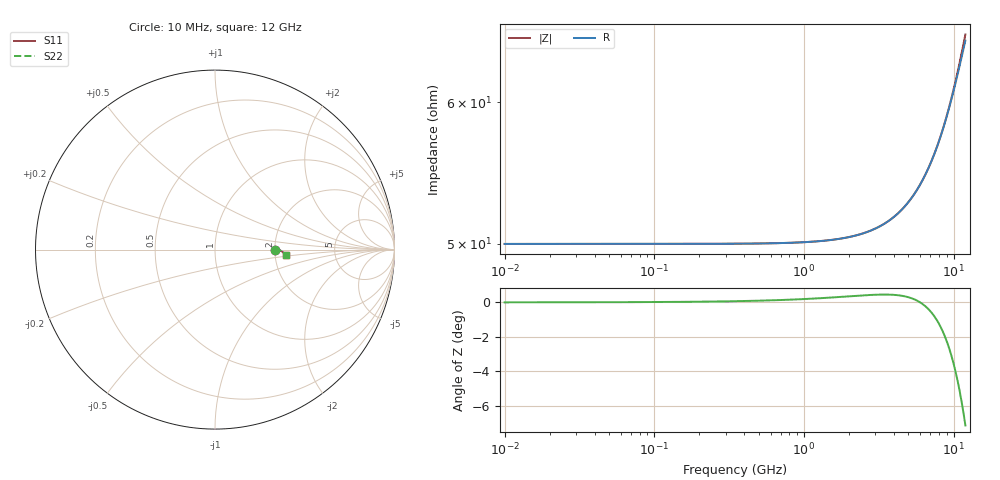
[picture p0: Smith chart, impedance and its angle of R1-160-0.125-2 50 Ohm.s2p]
!version-2
!date-03.2021
# MHz S RI R 50
!Freq ReS11 ImS11 ReS21 ImS21 ReS12 ImS12 ReS22 ImS22
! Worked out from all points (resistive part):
!   601 points, 10 MHz to 12 GHz, reference 50 ohm
!   read as one part in series: R = 50 ohm at 70 MHz
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10  0.3333 7.68e-06  0.6667 -7.7e-06  0.6667 -7.7e-06  0.3333 7.67e-06
510  0.3335 0.000389  0.6665 -0.00039  0.6665 -0.00039  0.3335 0.000388
1010  0.3338 0.000754  0.6662 -0.000755  0.6662 -0.000755  0.3338 0.000753
1510  0.3345 0.00109  0.6655 -0.00109  0.6655 -0.00109  0.3345 0.00109
2010  0.3353 0.00137  0.6647 -0.00138  0.6647 -0.00138  0.3353 0.00137
2510  0.3364 0.00159  0.6636 -0.0016  0.6636 -0.0016  0.3364 0.00159
3010  0.3378 0.00174  0.6622 -0.00174  0.6622 -0.00174  0.3378 0.00173
3510  0.3393 0.00178  0.6607 -0.00179  0.6607 -0.00179  0.3393 0.00178
4010  0.3412 0.00171  0.6588 -0.00172  0.6588 -0.00172  0.3412 0.00171
4490  0.3431 0.00152  0.6569 -0.00153  0.6569 -0.00153  0.3431 0.00152
4990  0.3454 0.00118  0.6546 -0.00119  0.6546 -0.00119  0.3454 0.00118
6010  0.3507 -5.13e-05  0.6493 4.37e-05  0.6493 4.37e-05  0.3507 -5.65e-05
7030  0.3568 -0.00214  0.6432 0.00213  0.6432 0.00213  0.3568 -0.00214
8010  0.3634 -0.00509  0.6366 0.00508  0.6366 0.00508  0.3634 -0.0051
8530  0.3672 -0.0071  0.6328 0.00709  0.6328 0.00709  0.3672 -0.0071
9030  0.371 -0.00933  0.629 0.00932  0.629 0.00932  0.371 -0.00934
9530  0.3749 -0.0119  0.6251 0.0119  0.6251 0.0119  0.3749 -0.0119
10010  0.3787 -0.0147  0.6213 0.0147  0.6213 0.0147  0.3787 -0.0147
10490  0.3826 -0.0178  0.6174 0.0178  0.6174 0.0178  0.3826 -0.0178
10970  0.3866 -0.0212  0.6134 0.0212  0.6134 0.0212  0.3866 -0.0213
11410  0.3903 -0.0247  0.6097 0.0247  0.6097 0.0247  0.3903 -0.0247
12000  0.3952 -0.0299  0.6048 0.0299  0.6048 0.0299  0.3952 -0.0299
